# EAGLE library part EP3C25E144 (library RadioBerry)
EP3C25E144 edit this description Auto generated by make-symbol-device-package-bsdl.ulp Rev. 20 Source: EP3C25E144.bsd http://www.altera.com/support/devices/bsdl/cyclone3/cyc3-index.jsp
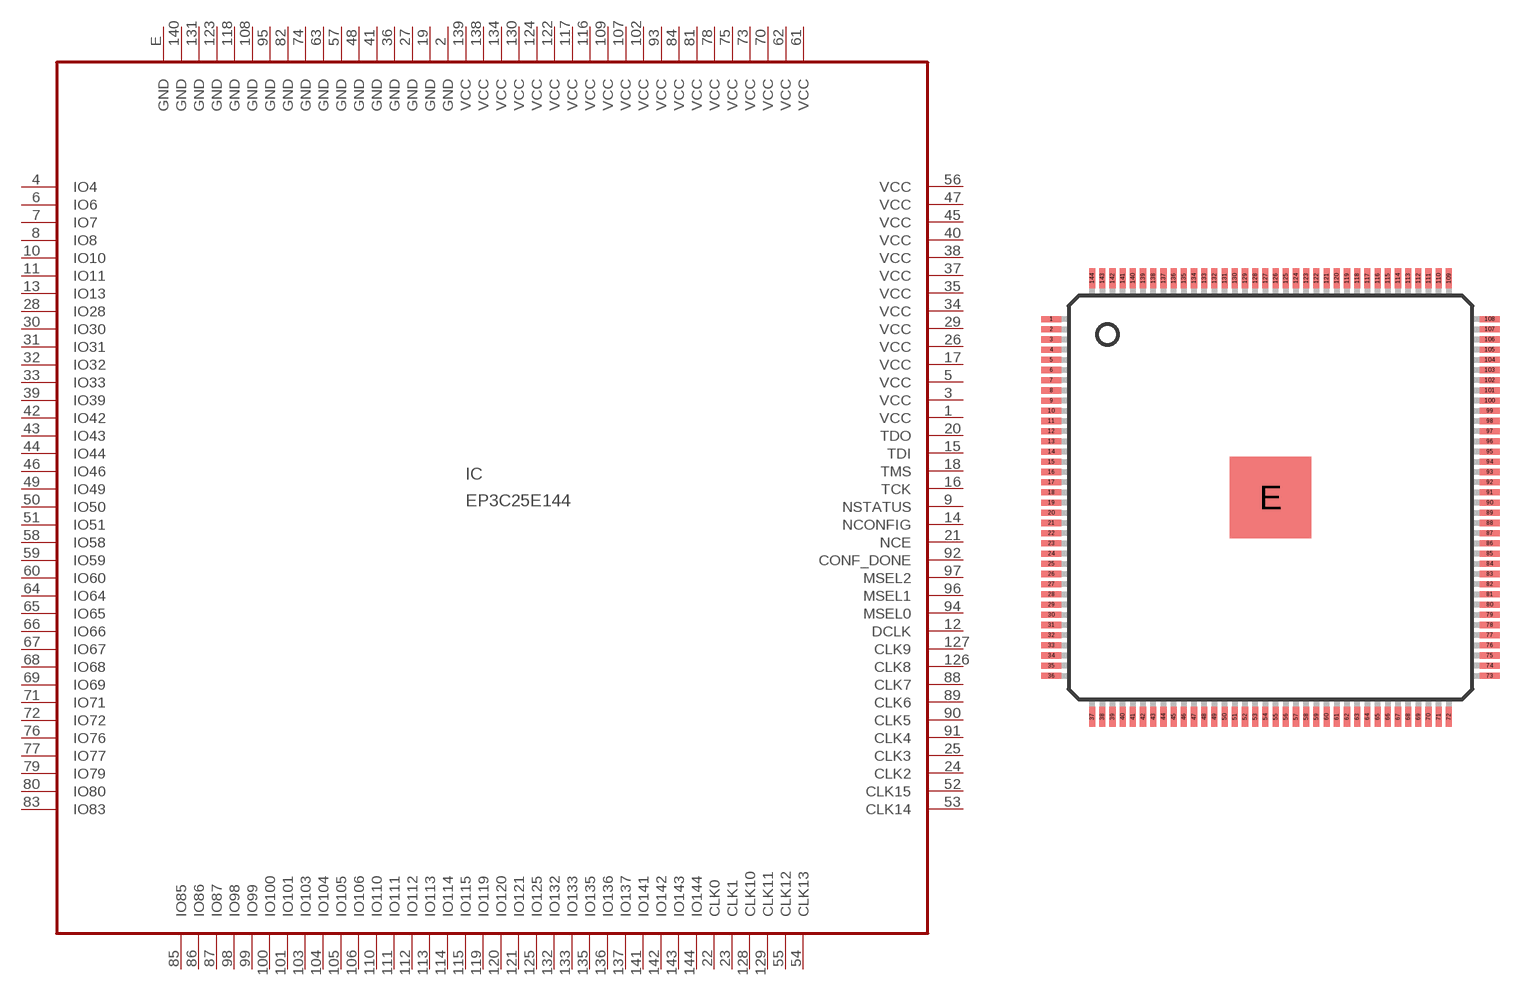
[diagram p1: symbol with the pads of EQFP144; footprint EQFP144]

Designator prefix IC

## EP3C25E144 (MPN: EP3C25E144C8N; OC_FARNELL: 1453474; OC_NEWARK: 51R0605)  [EQFP144]
1  VCC  pwr
2  GND  pwr
3  VCC  pwr
4  IO4  pas
5  VCC  pwr
6  IO6  pas
7  IO7  out
8  IO8  out
9  NSTATUS  in
10  IO10
11  IO11
12  DCLK  in
13  IO13
14  NCONFIG  in
15  TDI  in
16  TCK  in
17  VCC  pwr
18  TMS  in
19  GND  pwr
20  TDO  out
21  NCE  in
22  CLK0  in
23  CLK1  in
24  CLK2  in
25  CLK3  in
26  VCC  pwr
27  GND  pwr
28  IO28
29  VCC  pwr
30  IO30
31  IO31
32  IO32
33  IO33
34  VCC  pwr
35  VCC  pwr
36  GND  pwr
37  VCC  pwr
38  VCC  pwr
39  IO39
40  VCC  pwr
41  GND  pwr
42  IO42
43  IO43
44  IO44
45  VCC  pwr
46  IO46
47  VCC  pwr
48  GND  pwr
49  IO49
50  IO50
51  IO51
52  CLK15  in
53  CLK14  in
54  CLK13  in
55  CLK12  in
56  VCC  pwr
57  GND  pwr
58  IO58
59  IO59
60  IO60
61  VCC  pwr
62  VCC  pwr
63  GND  pwr
64  IO64
65  IO65
66  IO66
67  IO67
68  IO68
69  IO69
70  VCC  pwr
71  IO71
72  IO72
73  VCC  pwr
74  GND  pwr
75  VCC  pwr
76  IO76
77  IO77
78  VCC  pwr
79  IO79
80  IO80
81  VCC  pwr
82  GND  pwr
83  IO83
84  VCC  pwr
85  IO85
86  IO86
87  IO87
88  CLK7  in
89  CLK6  in
90  CLK5  in
91  CLK4  in
92  CONF_DONE  in
93  VCC  pwr
94  MSEL0  in
95  GND  pwr
96  MSEL1  in
97  MSEL2  in
98  IO98
99  IO99
100  IO100
101  IO101
102  VCC  pwr
103  IO103
104  IO104
105  IO105
106  IO106
107  VCC  pwr
108  GND  pwr
109  VCC  pwr
110  IO110
111  IO111
112  IO112
113  IO113
114  IO114
115  IO115
116  VCC  pwr
117  VCC  pwr
118  GND  pwr
119  IO119
120  IO120
121  IO121
122  VCC  pwr
123  GND  pwr
124  VCC  pwr
125  IO125
126  CLK8  in
127  CLK9  in
128  CLK10  in
129  CLK11  in
130  VCC  pwr
131  GND  pwr
132  IO132
133  IO133
134  VCC  pwr
135  IO135
136  IO136
137  IO137
138  VCC  pwr
139  VCC  pwr
140  GND  pwr
141  IO141
142  IO142
143  IO143
144  IO144
E  GND  pwr

## Footprint EQFP144 (pad centres in mm)
EQFP144 Source: http://www.altera.com/literature/ds/144-EQFP.pdf
smd 1 x 0.3: 1 -10.75,8.75; 2 -10.75,8.25; 3 -10.75,7.75; 4 -10.75,7.25; 5 -10.75,6.75; 6 -10.75,6.25; 7 -10.75,5.75; 8 -10.75,5.25; 9 -10.75,4.75; 10 -10.75,4.25; 11 -10.75,3.75; 12 -10.75,3.25; 13 -10.75,2.75; 14 -10.75,2.25; 15 -10.75,1.75; 16 -10.75,1.25; 17 -10.75,0.75; 18 -10.75,0.25; 19 -10.75,-0.25; 20 -10.75,-0.75; 21 -10.75,-1.25; 22 -10.75,-1.75; 23 -10.75,-2.25; 24 -10.75,-2.75; 25 -10.75,-3.25; 26 -10.75,-3.75; 27 -10.75,-4.25; 28 -10.75,-4.75; 29 -10.75,-5.25; 30 -10.75,-5.75; 31 -10.75,-6.25; 32 -10.75,-6.75; 33 -10.75,-7.25; 34 -10.75,-7.75; 35 -10.75,-8.25; 36 -10.75,-8.75; 73 10.75,-8.75; 74 10.75,-8.25; 75 10.75,-7.75; 76 10.75,-7.25; 77 10.75,-6.75; 78 10.75,-6.25; 79 10.75,-5.75; 80 10.75,-5.25; 81 10.75,-4.75; 82 10.75,-4.25; 83 10.75,-3.75; 84 10.75,-3.25; 85 10.75,-2.75; 86 10.75,-2.25; 87 10.75,-1.75; 88 10.75,-1.25; 89 10.75,-0.75; 90 10.75,-0.25; 91 10.75,0.25; 92 10.75,0.75; 93 10.75,1.25; 94 10.75,1.75; 95 10.75,2.25; 96 10.75,2.75; 97 10.75,3.25; 98 10.75,3.75; 99 10.75,4.25; 100 10.75,4.75; 101 10.75,5.25; 102 10.75,5.75; 103 10.75,6.25; 104 10.75,6.75; 105 10.75,7.25; 106 10.75,7.75; 107 10.75,8.25; 108 10.75,8.75
smd 0.3 x 1: 37 -8.75,-10.75; 38 -8.25,-10.75; 39 -7.75,-10.75; 40 -7.25,-10.75; 41 -6.75,-10.75; 42 -6.25,-10.75; 43 -5.75,-10.75; 44 -5.25,-10.75; 45 -4.75,-10.75; 46 -4.25,-10.75; 47 -3.75,-10.75; 48 -3.25,-10.75; 49 -2.75,-10.75; 50 -2.25,-10.75; 51 -1.75,-10.75; 52 -1.25,-10.75; 53 -0.75,-10.75; 54 -0.25,-10.75; 55 0.25,-10.75; 56 0.75,-10.75; 57 1.25,-10.75; 58 1.75,-10.75; 59 2.25,-10.75; 60 2.75,-10.75; 61 3.25,-10.75; 62 3.75,-10.75; 63 4.25,-10.75; 64 4.75,-10.75; 65 5.25,-10.75; 66 5.75,-10.75; 67 6.25,-10.75; 68 6.75,-10.75; 69 7.25,-10.75; 70 7.75,-10.75; 71 8.25,-10.75; 72 8.75,-10.75; 109 8.75,10.75; 110 8.25,10.75; 111 7.75,10.75; 112 7.25,10.75; 113 6.75,10.75; 114 6.25,10.75; 115 5.75,10.75; 116 5.25,10.75; 117 4.75,10.75; 118 4.25,10.75; 119 3.75,10.75; 120 3.25,10.75; 121 2.75,10.75; 122 2.25,10.75; 123 1.75,10.75; 124 1.25,10.75; 125 0.75,10.75; 126 0.25,10.75; 127 -0.25,10.75; 128 -0.75,10.75; 129 -1.25,10.75; 130 -1.75,10.75; 131 -2.25,10.75; 132 -2.75,10.75; 133 -3.25,10.75; 134 -3.75,10.75; 135 -4.25,10.75; 136 -4.75,10.75; 137 -5.25,10.75; 138 -5.75,10.75; 139 -6.25,10.75; 140 -6.75,10.75; 141 -7.25,10.75; 142 -7.75,10.75; 143 -8.25,10.75; 144 -8.75,10.75
smd 4 x 4: E 0,0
